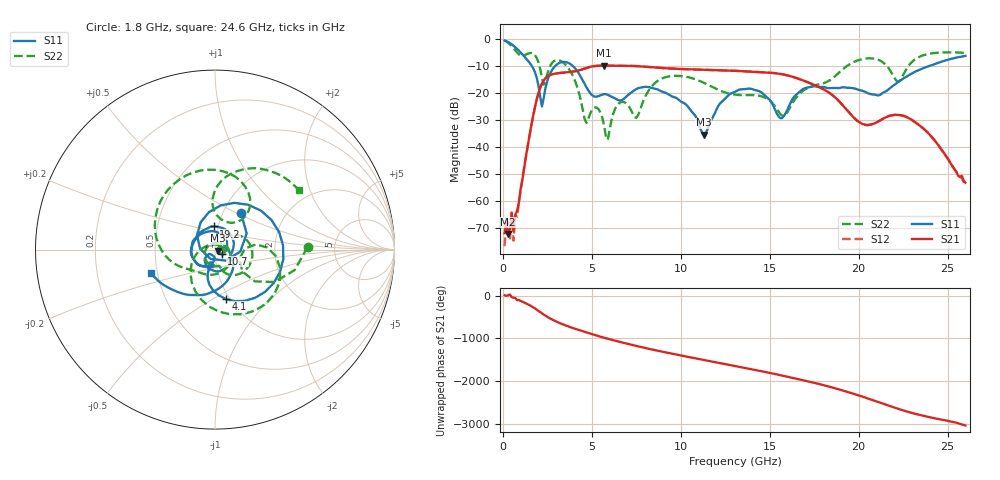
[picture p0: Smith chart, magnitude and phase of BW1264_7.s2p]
!Keysight Technologies,N5245B,MY57181159,A.13.60.06
!Date: Friday, December 18, 2020 23:52:16
!Correction: S11(Full 2 Port(1,2))
!S21(Full 2 Port(1,2))
!S12(Full 2 Port(1,2))
!S22(Full 2 Port(1,2))
!S2P File: Measurements: S11, S21, S12, S22:
# Hz S  dB  R 50
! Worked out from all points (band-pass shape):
!   260 points, 100 MHz to 26 GHz, reference 50 ohm
!   highest |S21| = -9.69 dB at 5.7 GHz (marker M1); lowest = -72.2 dB at 300 MHz (marker M2)
!   |S21| within 3 dB of the highest: 2.921 GHz to 15.51 GHz (12.59 GHz wide, 137 % of centre)
!   lowest |S11| = -35.3 dB at 11.3 GHz (marker M3), VSWR 1.03, Z = 51.6 - j0.652 ohm
!   |S11| at or under -10 dB: 1.643 GHz to 2.921 GHz (1.278 GHz wide, 56 % of centre); 3.962 GHz to 23.9 GHz (19.94 GHz wide, 143 % of centre)
!   |S22| runs from -37.2 to -0.4 dB; largest |S21 - S12| = 0.00053
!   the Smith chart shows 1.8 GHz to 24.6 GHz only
!   S11 on the Smith chart (normalised r, x): 1.8 GHz: 1.21, +0.53; 4.1 GHz: 0.96, -0.57; 10.7 GHz: 1.07, -0.05; 19.2 GHz: 0.96, +0.25; 24.6 GHz: 0.46, -0.14
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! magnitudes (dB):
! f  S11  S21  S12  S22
! 100 MHz  -0.4  -71.8  -76.7  -0.4
! 300 MHz  -1.0  -72.2  -68.0  -1.3
! 400 MHz  -1.3  -70.2  -74.4  -1.8
! 500 MHz  -1.8  -64.5  -64.1  -2.5
! 600 MHz  -2.3  -71.1  -74.6  -3.2
! 1.8 GHz  -12.1  -25.3  -25.2  -5.7
! 2.2 GHz  -24.8  -16.4  -16.3  -14.2
! 2.9 GHz  -10.1  -12.7  -12.7  -7.9
! 4.1 GHz  -11.0  -11.7  -11.7  -16.1
! 4.5 GHz  -15.3  -11.0  -11.0  -26.3
! 5.7 GHz  -20.3  -9.7  -9.7  -32.3
! 7.5 GHz  -18.4  -9.9  -9.9  -29.1
! 8.8 GHz  -18.9  -10.5  -10.5  -15.0
! 10.7 GHz  -27.4  -11.1  -11.1  -14.5
! 11.3 GHz  -35.3  -11.2  -11.2  -16.1
! 13.1 GHz  -19.2  -11.6  -11.6  -20.5
! 15.6 GHz  -29.2  -12.8  -12.8  -27.7
! 17.4 GHz  -17.4  -16.6  -16.6  -17.3
! 19.2 GHz  -17.8  -25.1  -25.1  -10.5
! 21.7 GHz  -18.4  -28.4  -28.4  -10.8
! 24.6 GHz  -8.4  -40.3  -40.3  -4.8
! 26 GHz  -6.1  -53.1  -53.0  -5.0
